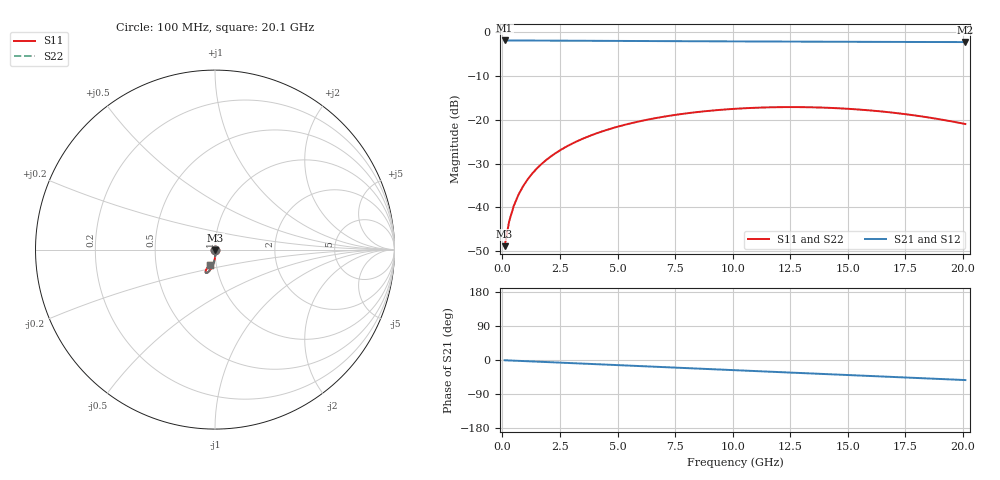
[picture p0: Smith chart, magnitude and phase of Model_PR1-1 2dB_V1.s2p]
!version-1
!date-07.2020
!Series
#	GHZ S RI R 50.0
!	FREQ.GHZ	S11RE	S11IM	S21RE	S21IM	S12RE	S12IM	S22RE	S22IM
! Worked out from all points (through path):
!   101 points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, 100 MHz to 20.1 GHz, reference 50 ohm
!   highest |S21| = -1.97 dB at 100 MHz (marker M1); lowest = -2.3 dB at 20.1 GHz (marker M2)
!   group delay of S21, straight-line fit = 7.27 ps
!   lowest |S11| = -48.8 dB at 100 MHz (marker M3), VSWR 1.01, Z = 50.2 - j0.312 ohm
!   |S11| at or under -10 dB: start of sweep to end of sweep
!   |S22| runs from -48.8 to -17.1 dB; largest |S21 - S12| = 0
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0.1  0.00187 -0.00311  0.7972 -0.00946  0.7972 -0.00946  0.00187 -0.00311
0.3  0.00213 -0.00666  0.7968 -0.0166  0.7968 -0.0166  0.00213 -0.00666
0.5  0.00231 -0.0102  0.7963 -0.0238  0.7963 -0.0238  0.00231 -0.0102
0.7  0.00241 -0.0137  0.7957 -0.0309  0.7957 -0.0309  0.00241 -0.0137
0.9  0.00242 -0.0173  0.795 -0.0381  0.795 -0.0381  0.00242 -0.0173
1.1  0.00235 -0.0208  0.7943 -0.0453  0.7943 -0.0453  0.00235 -0.0208
1.5  0.002 -0.0277  0.7925 -0.0596  0.7925 -0.0596  0.002 -0.0277
2.1  0.000945 -0.038  0.7895 -0.0811  0.7895 -0.0811  0.000945 -0.038
2.7  -0.000662 -0.0479  0.7857 -0.1025  0.7857 -0.1025  -0.000662 -0.0479
3.5  -0.00354 -0.0607  0.7798 -0.1309  0.7798 -0.1309  -0.00354 -0.0607
4.3  -0.00712 -0.0726  0.7729 -0.1591  0.7729 -0.1591  -0.00712 -0.0726
5.1  -0.0112 -0.0837  0.7649 -0.187  0.7649 -0.187  -0.0112 -0.0837
5.9  -0.0157 -0.0937  0.7559 -0.2146  0.7559 -0.2146  -0.0157 -0.0937
6.9  -0.0216 -0.1046  0.7433 -0.2485  0.7433 -0.2485  -0.0216 -0.1046
8.5  -0.0311 -0.1182  0.7202 -0.3013  0.7202 -0.3013  -0.0311 -0.1182
10.1  -0.0399 -0.1267  0.6937 -0.3519  0.6937 -0.3519  -0.0399 -0.1267
11.7  -0.0468 -0.1301  0.6638 -0.4002  0.6638 -0.4002  -0.0468 -0.1301
13.5  -0.0516 -0.128  0.6266 -0.4514  0.6266 -0.4514  -0.0516 -0.128
15.3  -0.0521 -0.1206  0.5857 -0.4993  0.5857 -0.4993  -0.0521 -0.1206
16.9  -0.0482 -0.1104  0.5464 -0.5389  0.5464 -0.5389  -0.0482 -0.1104
18.5  -0.0399 -0.0981  0.5045 -0.5759  0.5045 -0.5759  -0.0399 -0.0981
20.1  -0.0266 -0.0851  0.4601 -0.6103  0.4601 -0.6103  -0.0266 -0.0851
